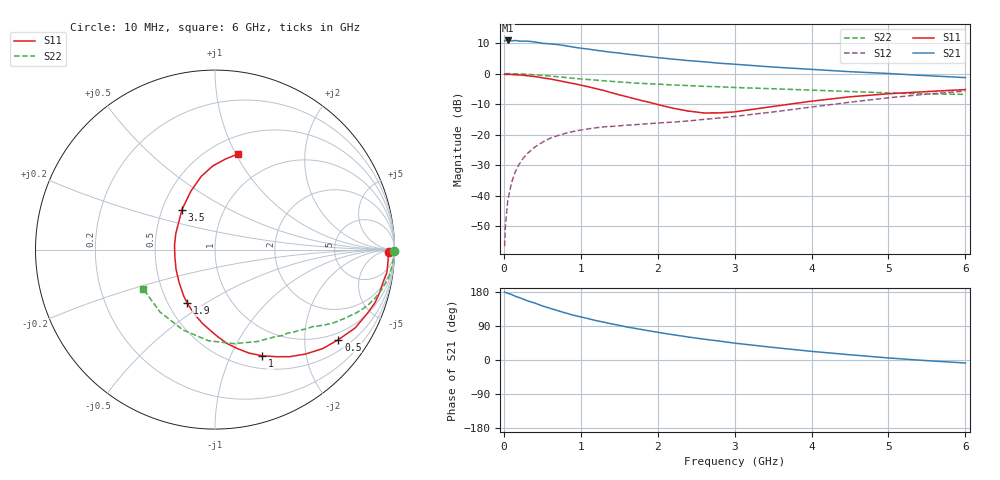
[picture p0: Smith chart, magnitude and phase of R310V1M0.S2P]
! SIEMENS Small Signal Semiconductors
! BFR181
! Si NPN RF Bipolar Junction Transistor in SOT23
! VCE = 10 V  IC = 1 mA
! Common Emitter S-Parameters:  May  1996
# GHz  S  MA  R  50
!  f  S11  S21  S12  S22
! GHz  MAG  ANG  MAG  ANG  MAG  ANG  MAG  ANG
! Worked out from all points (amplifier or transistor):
!   36 points, 10 MHz to 6 GHz, reference 50 ohm
!   highest |S21| = 10.8 dB at 50 MHz (marker M1)
!   |S21| within 3 dB of that: start of sweep to 1.145 GHz
!   unconditionally stable (mu >= 1): 2.09 GHz to 3.731 GHz
!   at 250 MHz: K = 0.16, MSG = 19.2 dB, |S12| = -27.7 dB
!   at 1.4 GHz: K = 0.75, MSG = 12.1 dB, |S12| = -17.3 dB
!   at 6 GHz: K = 0.87, MSG = 2.2 dB, |S12| = -5.7 dB
!   S11 on the Smith chart (normalised r, x): 10 MHz: 53, -23; 500 MHz: 0.79, -2.87; 1 GHz: 0.65, -1.33; 1.9 GHz: 0.62, -0.42; 3.5 GHz: 0.63, +0.31; 6 GHz: 0.67, +1.02
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0.01  0.9686 -0.8  3.408 179.3  0.0015 87.8  0.9979 -0.4
0.02  0.9656 -1.2  3.465 178.2  0.0032 89.5  0.9916 -0.7
0.05  0.9664 -3.8  3.476 176.2  0.0082 87.3  0.9971 -1.8
0.1  0.9662 -7.6  3.42 172.8  0.0164 85.5  0.9938 -3.5
0.15  0.9541 -10.9  3.471 168.1  0.025 81.5  0.9893 -5.5
0.2  0.9482 -14.6  3.4 164.7  0.0329 80.3  0.9849 -7.1
0.3  0.9213 -22.5  3.391 156.8  0.0485 75.8  0.9722 -10.6
0.4  0.8946 -29.2  3.291 150.4  0.0623 70.9  0.953 -13.8
0.5  0.8512 -36.1  3.123 142.8  0.0751 67.1  0.9326 -16.8
0.7  0.7707 -49.0  2.976 130.3  0.0964 60.0  0.8854 -22.0
0.8  0.7273 -55.1  2.853 124.2  0.1052 56.7  0.8614 -24.2
1  0.6479 -66.0  2.598 113.7  0.1189 52.0  0.8163 -28.1
1.1  0.6063 -71.9  2.508 109.0  0.1245 50.3  0.7971 -29.7
1.3  0.528 -82.6  2.312 99.8  0.1341 47.2  0.7617 -32.8
1.6  0.4175 -99.6  2.076 87.1  0.143 45.0  0.7151 -36.6
1.9  0.3361 -117.5  1.884 76.6  0.1516 44.7  0.6791 -40.2
2.2  0.2705 -137.8  1.72 66.7  0.1606 45.8  0.6498 -43.8
3  0.2358 157.9  1.42 44.5  0.199 49.9  0.5908 -55.1
3.5  0.2894 129.5  1.276 33.2  0.2354 50.9  0.5637 -65.3
4.5  0.4162 100.5  1.072 13.8  0.3395 47.2  0.5088 -94.2
5.5  0.5068 83.6  0.923 -1.7  0.4606 35.5  0.4636 -131.2
6  0.5464 76.7  0.858 -7.9  0.5169 28.0  0.4562 -151.4
